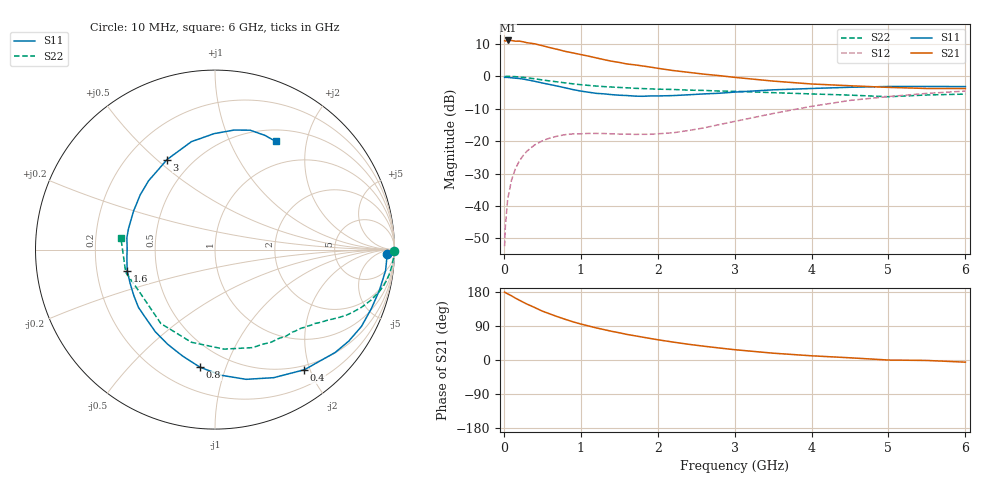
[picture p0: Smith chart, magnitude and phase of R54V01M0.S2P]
! SIEMENS Small Signal Semiconductors
! BFR183
! Si NPN RF Bipolar Junction Transistor in SOT23
! VCE = 4 V  IC = 1 mA
! Common Emitter S-Parameters:  May  1996
# GHz  S  MA  R  50
!  f  S11  S21  S12  S22
! GHz  MAG  ANG  MAG  ANG  MAG  ANG  MAG  ANG
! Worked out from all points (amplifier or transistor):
!   36 points, 10 MHz to 6 GHz, reference 50 ohm
!   highest |S21| = 11.0 dB at 50 MHz (marker M1)
!   |S21| within 3 dB of that: start of sweep to 737.9 MHz
!   unconditionally stable (mu >= 1): 1.662 GHz to 2.947 GHz
!   at 250 MHz: K = 0.16, MSG = 17.5 dB, |S12| = -24.5 dB
!   at 1.4 GHz: K = 0.85, MSG = 11.2 dB, |S12| = -17.8 dB
!   at 6 GHz: K = 0.95, MSG = 0.4 dB, |S12| = -4.6 dB
!   S11 on the Smith chart (normalised r, x): 10 MHz: 35, -20; 400 MHz: 0.43, -1.91; 800 MHz: 0.35, -0.82; 1.6 GHz: 0.33, -0.10; 3 GHz: 0.36, +0.54; 6 GHz: 0.65, +1.50
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0.01  0.9579 -1.4  3.516 179.3  0.0024 92.5  0.9994 -0.5
0.02  0.9586 -2.8  3.474 177.7  0.0049 89.9  0.9871 -1.0
0.05  0.9576 -7.0  3.552 174.6  0.0127 85.5  0.9969 -2.5
0.1  0.9439 -13.8  3.545 169.4  0.0251 81.2  0.9899 -5.1
0.15  0.9311 -20.7  3.459 163.3  0.0374 77.7  0.983 -7.5
0.2  0.9214 -27.7  3.47 158.0  0.0489 73.5  0.9729 -9.9
0.25  0.9029 -34.4  3.388 152.7  0.0596 69.3  0.9596 -12.3
0.4  0.8342 -53.4  3.154 138.6  0.0871 59.3  0.912 -18.1
0.5  0.7848 -65.4  2.953 129.0  0.1009 53.2  0.8763 -21.6
0.7  0.7017 -86.9  2.582 114.1  0.1195 43.7  0.8162 -26.7
0.8  0.6609 -97.2  2.408 107.2  0.1256 39.9  0.7873 -28.7
0.9  0.6205 -106.8  2.281 100.7  0.129 37.1  0.7617 -30.5
1.1  0.566 -125.9  2.037 89.9  0.1312 33.1  0.7211 -33.9
1.3  0.5345 -142.9  1.801 80.3  0.1308 31.1  0.6907 -36.6
1.6  0.5031 -166.6  1.541 67.5  0.1277 31.5  0.6619 -40.8
1.9  0.4955 172.4  1.384 56.9  0.1272 37.7  0.6374 -45.4
2.2  0.5021 154.6  1.222 47.3  0.1341 44.5  0.6241 -50.5
3  0.5684 118.1  0.959 27.2  0.2008 57.5  0.585 -69.0
3.5  0.6157 102.3  0.84 18.0  0.2659 56.4  0.5567 -84.8
4.5  0.6746 80.9  0.712 5.8  0.4232 43.3  0.5106 -126.2
5.5  0.6946 66.4  0.646 -1.2  0.5429 26.2  0.5134 -165.7
6  0.6912 60.7  0.645 -5.7  0.5893 16.1  0.5289 172.7
